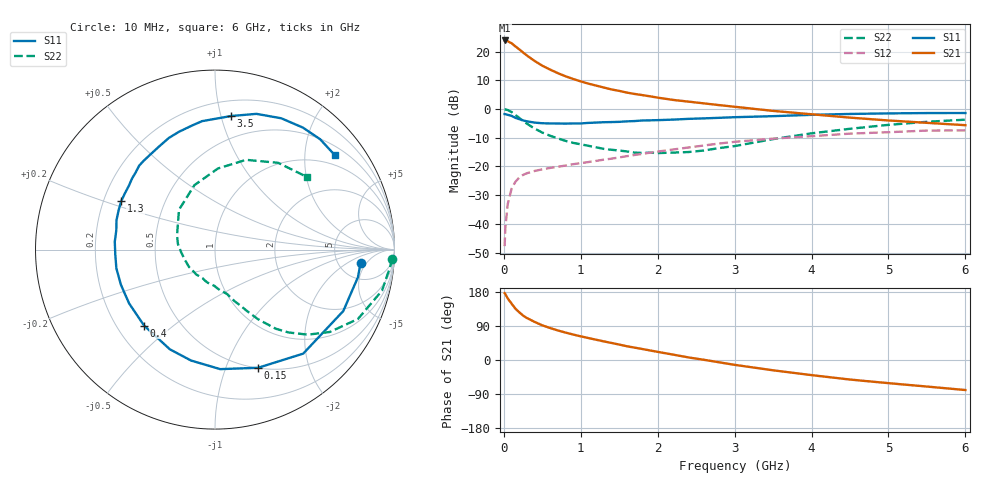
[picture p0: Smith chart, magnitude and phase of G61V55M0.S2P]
! SIEMENS Small Signal Semiconductors
! BFG193
! Si NPN RF Bipolar Junction Transistor in SOT223
! VCE = 1.5 V  IC = 5 mA
! Common Emitter S-Parameters:  August  1996
# GHz  S  MA  R  50
!  f  S11  S21  S12  S22
! GHz  MAG  ANG  MAG  ANG  MAG  ANG  MAG  ANG
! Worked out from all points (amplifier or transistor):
!   36 points, 10 MHz to 6 GHz, reference 50 ohm
!   highest |S21| = 23.8 dB at 10 MHz (marker M1)
!   |S21| within 3 dB of that: start of sweep to 195.8 MHz
!   unconditionally stable (mu >= 1): 1.085 GHz to 2.784 GHz
!   at 250 MHz: K = 0.35, MSG = 21.3 dB, |S12| = -23.0 dB
!   at 1.4 GHz: K = 1.09, MAG = 10.2 dB, |S12| = -17.3 dB
!   at 6 GHz: K = 0.94, MSG = 0.9 dB, |S12| = -7.4 dB
!   S11 on the Smith chart (normalised r, x): 10 MHz: 8.13, -3.63; 150 MHz: 0.50, -1.30; 400 MHz: 0.31, -0.40; 1.3 GHz: 0.27, +0.22; 3.5 GHz: 0.32, +1.08; 6 GHz: 0.72, +2.73
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0.01  0.8142 -5.3  15.57 176.4  0.0041 91.0  0.9885 -2.9
0.02  0.8113 -10.9  15.55 173.8  0.0087 87.9  0.9804 -5.7
0.05  0.7924 -25.6  15.11 162.6  0.0219 76.8  0.9581 -13.8
0.1  0.7599 -49.7  13.93 149.0  0.0407 66.4  0.8853 -25.9
0.15  0.7008 -70.0  12.28 135.5  0.054 56.5  0.7867 -35.7
0.2  0.6666 -87.5  10.91 126.0  0.064 50.3  0.7015 -42.5
0.25  0.6323 -102.2  9.618 117.3  0.0712 45.4  0.6174 -48.4
0.3  0.6097 -114.4  8.519 110.7  0.0762 42.4  0.5554 -52.5
0.4  0.5792 -133.0  6.856 100.5  0.0834 38.0  0.4554 -58.3
0.5  0.5647 -148.0  5.663 91.5  0.0891 35.4  0.3887 -62.3
0.6  0.5596 -159.6  4.853 84.5  0.0942 34.9  0.3427 -65.6
0.7  0.5593 -169.3  4.216 78.1  0.0985 34.4  0.3085 -69.1
0.9  0.5601 175.5  3.333 67.2  0.1094 34.4  0.2576 -74.6
1.1  0.5725 163.5  2.759 57.9  0.1193 34.5  0.2285 -82.7
1.3  0.5882 152.8  2.359 49.1  0.1314 34.4  0.202 -90.9
1.6  0.6089 139.3  1.926 36.3  0.1512 32.8  0.1824 -107.3
2.2  0.6532 118.6  1.438 14.2  0.1974 26.7  0.1741 -146.5
2.8  0.7017 100.9  1.168 -6.1  0.2506 17.1  0.2089 171.4
3.5  0.7498 83.1  0.926 -27.2  0.3047 1.9  0.2992 132.1
4.5  0.8196 63.2  0.707 -51.6  0.3725 -18.0  0.4523 87.9
5.5  0.8492 46.4  0.574 -70.1  0.421 -42.4  0.5983 53.9
6  0.8502 38.1  0.522 -79.3  0.4242 -56.2  0.6517 38.5
